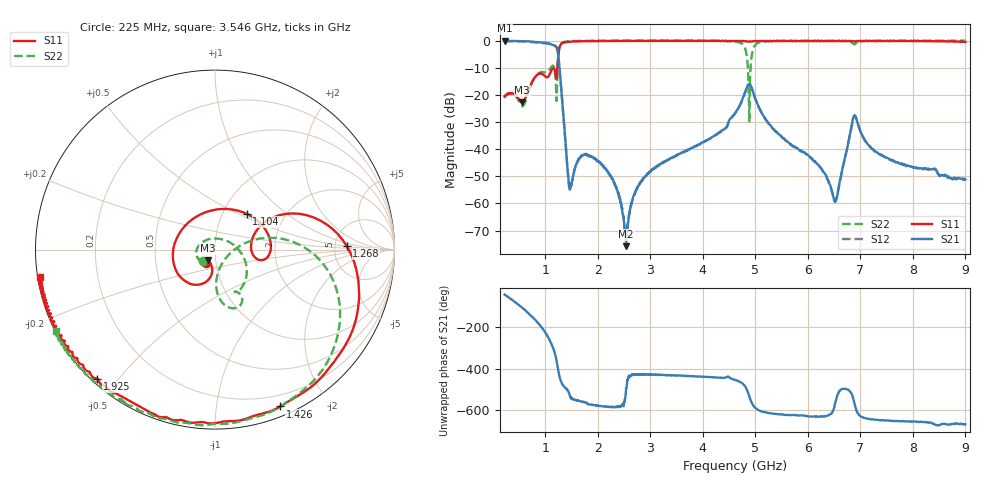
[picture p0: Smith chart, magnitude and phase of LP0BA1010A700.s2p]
!Agilent Technologies,E8358A,US41080443,A.07.50.56
!Agilent E8358A: A.07.50.56
!Date: Monday, May 09, 2016 11:51:35
!Correction: S11(Full 2 Port(1,2))
!S21(Full 2 Port(1,2))
!S12(Full 2 Port(1,2))
!S22(Full 2 Port(1,2))
!S2P File: Measurements: S11, S21, S12, S22:Log Frequency Sweep
# Hz S  dB  R 50
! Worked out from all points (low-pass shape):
!   1601 points, 225 MHz to 9 GHz, reference 50 ohm
!   highest |S21| = -0.05 dB at 230.8 MHz (marker M1); lowest = -75.8 dB at 2.538 GHz (marker M2)
!   |S21| within 3 dB of the highest: start of sweep to 1.226 GHz
!   lowest |S11| = -22.7 dB at 560.7 MHz (marker M3), VSWR 1.16, Z = 45.7 - j5.53 ohm
!   |S11| at or under -10 dB: start of sweep to 1.229 GHz
!   |S22| runs from -30.1 to 0.1 dB; largest |S21 - S12| = 0.02
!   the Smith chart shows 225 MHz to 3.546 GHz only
!   S11 on the Smith chart (normalised r, x): 225 MHz: 0.89, -0.14; 1.104 GHz: 1.30, +0.56; 1.268 GHz: 6.47, +0.56; 1.426 GHz: 0.09, -1.50; 1.925 GHz: 0.02, -0.44; 3.546 GHz: 0.01, -0.08
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2.25e8  -20.67 -124.4  -0.05 -40.3  -0.21 -40.1  -20.55 -136.8
2.307792e8  -20.53 -125.1  -0.05 -41.3  -0.22 -41.1  -20.42 -138.1
5.606507e8  -22.74 -124.4  -0.16 -104.4  -0.32 -104.3  -24.11 97.7
8.829701e8  -12.24 -137.5  -0.63 175.6  -0.80 175.7  -11.87 -52.4
1.104259e9  -11.49 48.4  -1.28 86.4  -1.44 86.6  -9.92 -61.6
1.202593e9  -13.33 -8.5  -2.06 13.2  -2.23 13.4  -16.39 -85.9
1.268084e9  -2.69 1.6  -9.54 -76.4  -9.72 -76.2  -2.64 -21.2
1.42631e9  -0.48 -67.4  -48.26 -145.4  -48.23 -144.5  -0.26 -83.0
1.687749e9  -0.22 -103.0  -42.53 159.9  -42.72 160.6  -0.09 -114.0
1.92478e9  -0.23 -132.3  -43.24 142.5  -43.31 142.4  -0.08 -125.4
2.314644e9  -0.18 -148.8  -52.28 131.4  -52.49 133.1  -0.05 -136.9
2.538257e9  -0.07 -154.8  -75.76 -134.1  -73.21 -167.7  0.02 -141.2
3.152512e9  -0.13 -166.4  -46.03 -69.9  -46.05 -70.3  -0.02 -149.2
3.545866e9  -0.14 -171.2  -41.83 -74.5  -42.02 -74.5  -0.03 -153.1
4.622431e9  -0.10 178.2  -26.43 -95.7  -26.61 -95.6  -0.32 -175.4
4.907993e9  -0.30 175.0  -16.44 167.8  -16.60 168.4  -10.21 -93.2
5.199195e9  -0.17 172.3  -29.05 107.1  -29.23 106.7  -0.32 -153.0
6.081681e9  -0.11 160.4  -43.53 86.6  -43.67 86.5  -0.06 -178.5
6.517218e9  -0.09 156.7  -59.38 152.2  -59.37 147.8  -0.06 172.7
6.919835e9  -0.14 153.1  -28.45 120.0  -28.63 119.9  -0.88 170.6
7.553438e9  -0.16 149.2  -43.77 66.8  -43.85 67.1  -0.09 158.9
9e9  -0.48 131.6  -51.18 49.4  -50.95 51.6  0.04 147.7
